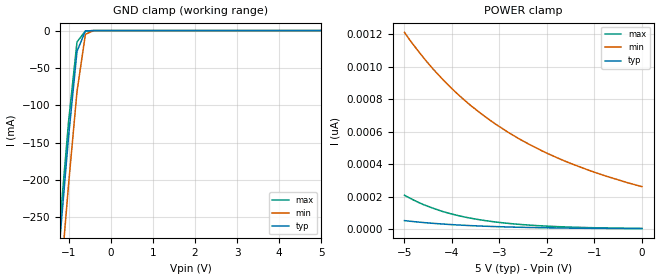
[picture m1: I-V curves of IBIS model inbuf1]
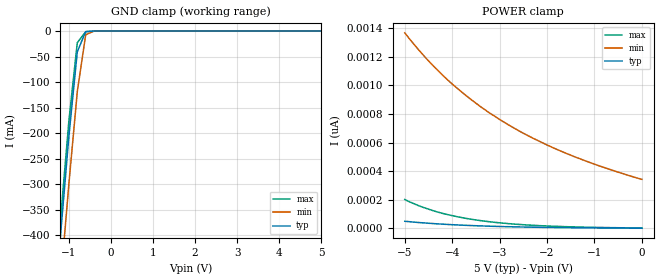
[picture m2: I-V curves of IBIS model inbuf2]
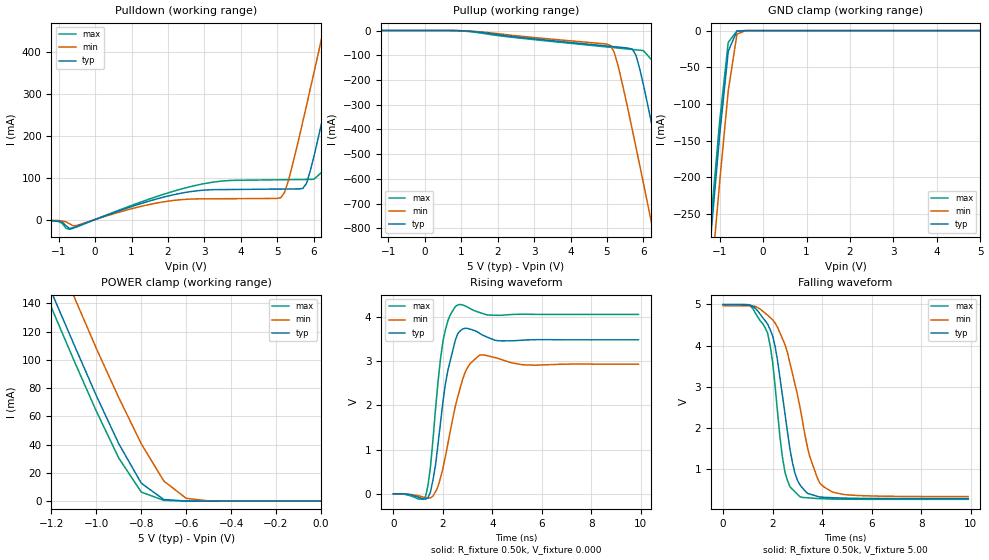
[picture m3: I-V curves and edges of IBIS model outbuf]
| IBIS file 66244l.ibs created by s2ibis2 version 1.0
| North Carolina State University Electronics Research Laboratory  1995
[IBIS ver]   2.1
[File name]   66244l.ibs
[File Rev]   0.1
[Date]   Friday, June 08, 2001
[Source]   IDT
[Notes]   1. Temp typ=25C, min=100C, max=0C 2. Ramp rates based on 500
   ohm load
[Copyright]   Copyright 2001, Integrated Device Technology, Inc.
[Disclaimer] Integrated Device Technology, Inc. ("IDT") hereby grants the
   user of this IBIS model a non-exclusive, nontransferable
   license to use this IBIS model under the following terms.
   The user is granted this license only to use the IBIS model
   and is not granted rights to sell, copy (except as needed to
   run the IBIS model), rent, lease or sub-license the IBIS model
   in whole or in part, or in modified form to anyone.
   The User may modify the IBIS model to suit its specific
   applications, but rights to derivative works and such
   modifications shall belong to IDT.
   This IBIS model is provided on an "AS IS" basis and IDT
   makes absolutely no warranty with respect to the information
   contained herein. IDT DISCLAIMS AND CUSTOMER WAIVES ALL
   WARRANTIES, EXPRESS AND IMPLIED, INCLUDING WARRANTIES OF
   MERCHANTABILITY AND FITNESS FOR A PARTICULAR PURPOSE. THE
   ENTIRE RISK AS TO QUALITY AND PERFORMANCE IS WITH THE
   USER ACCORDINGLY, IN NO EVENT SHALL IDT BE LIABLE
   FOR ANY DIRECT OR INDIRECT DAMAGES, WHETHER IN CONTRACT OR
   TORT, INCLUDING ANY LOST PROFITS OR OTHER INCIDENTAL,
   CONSEQUENTIAL, EXEMPLARY, OR PUNITIVE DAMAGES ARISING OUT OF
   THE USE OR APPLICATION OF THE IBIS model.  Further, IDT
   reserves the right to make changes without notice to any
   product herein to improve reliability, function, or design.
   IDT does not convey any license under patent rights or
   any other intellectual property rights, including those of
   third parties. IDT is not obligated to provide maintenance
   or support for the licensed IBIS model.
|   Component IDT54/74FCT166244T/AT/CT
[Component]   IDT54/74FCT166244T/AT/CT
[Manufacturer]   Integrated Device Technology Inc.
[Package]
| Following package parameters are for SO48-2(TSSOP) package
|[Package]
|| variable   typ   min   max
|R_pkg   15.00m   10.00m   20.00m
|L_pkg   2.30nh   1.40nh   4.50nH
|C_pkg   0.40pF   0.35pF   0.60pF
| Following package parameters are for SO48-1(SSOP), E48-1(CERPAK) packages
| variable   typ   min   max
R_pkg   15.00m   10.00m   20.00m
L_pkg   2.90nH   1.50nH   5.60nH
C_pkg   0.40pF   0.26pF   0.50pF
[Pin]  signal_name   model_name   R_pin   L_pin   C_pin
1   1OEB   inbuf1
2   1Y1   outbuf
3   1Y2   outbuf
4   GND   GND
5   1Y3   outbuf
6   1Y4   outbuf
7   VCC   POWER
8   2Y1   outbuf
9   2Y2   outbuf
10   GND   GND
11   2Y3   outbuf
12   2Y4   outbuf
13   3Y1   outbuf
14   3Y2   outbuf
15   GND   GND
16   3Y3   outbuf
17   3Y4   outbuf
18   VCC   POWER
19   4Y1   outbuf
20   4Y2   outbuf
21   GND   GND
22   4Y3   outbuf
23   4Y4   outbuf
24   4OEB   inbuf1
25   3OEB   inbuf1
26   4A4   inbuf2
27   4A3   inbuf2
28   GND   GND
29   4A2   inbuf2
30   4A1   inbuf2
31   VCC   POWER
32   3A4   inbuf2
33   3A3   inbuf2
34   GND   GND
35   3A2   inbuf2
36   3A1   inbuf2
37   2A4   inbuf2
38   2A3   inbuf2
39   GND   GND
40   2A2   inbuf2
41   2A1   inbuf2
42   VCC   POWER
43   1A4   inbuf2
44   1A3   inbuf2
45   GND   GND
46   1A2   inbuf2
47   1A1   inbuf2
48   2OEB   inbuf1
| Models and submodels in the file (3): inbuf1 (Input), inbuf2 (Input), outbuf (3-state)
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| in   IN1   dummy_model
| oe   OE1   dummy_model
|   Model inbuf1
[Model]   inbuf1
Model_type   Input
Vinl =  0.800V
Vinh =  2.000V
C_comp   3.00pF   NA   NA
[Temperature Range]   25.00   100.00   0.000
[Voltage Range]   5.00V   4.50V   5.50V
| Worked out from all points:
|   GND clamp passes 1 mA (typ) near -0.60 V on its own axis
[GND_clamp]
| voltage   I(typ)   I(min)   I(max)
-5V       -3.018A    -3.076A    -2.999A
-1.4V     -415mA     -480mA     -394mA
-1.2V     -276mA     -341mA     -255mA
-1V       -142mA     -206mA     -122mA
-800mV    -27.87mA   -81.82mA   -15.26mA
-600mV    -480uA     -4.848mA   -551uA
-400mV    -1.016uA   -20.86uA   -873nA
5V        1.855pA    303pA      2.085pA
[POWER_clamp]
| voltage   I(typ)   I(min)   I(max)
-5V       51.46pA    1.212nA    208pA
-4.6V     39.61pA    1.056nA    150pA
-4.4V     34.75pA    987pA      128pA
-4.1V     28.53pA    894pA      99.73pA
-3.9V     25.02pA    837pA      84.6pA
-3.6V     20.53pA    760pA      66.05pA
-3.1V     14.75pA    650pA      43.65pA
-2.8V     12.09pA    593pA      34.01pA
-2.4V     9.265pA    526pA      24.35pA
-1.7V     5.808pA    428pA      13.54pA
-800mV    3.178pA    330pA      6.324pA
0V        1.855pA    261pA      3.199pA
|   Model inbuf2
[Model]   inbuf2
Model_type   Input
Vinl =  0.800V
Vinh =  2.000V
C_comp   3.00pF   NA   NA
[Temperature Range]   25.00   100.00   0.000
[Voltage Range]   5.00V   4.50V   5.50V
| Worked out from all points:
|   GND clamp passes 1 mA (typ) near -0.60 V on its own axis
[GND_clamp]
| voltage   I(typ)   I(min)   I(max)
-5V       -4.387A    -4.471A    -4.36A
-1.4V     -604mA     -698mA     -573mA
-1.2V     -402mA     -496mA     -371mA
-1V       -207mA     -300mA     -177mA
-800mV    -40.8mA    -119mA     -22.8mA
-600mV    -973uA     -7.222mA   -1.303mA
-400mV    -6.41uA    -46.07uA   -11.93uA
5V        1.965pA    393pA      2.176pA
[POWER_clamp]
| voltage   I(typ)   I(min)   I(max)
-5V       50.2pA     1.366nA    202pA
-4.6V     38.73pA    1.207nA    146pA
-4.4V     34.01pA    1.136nA    124pA
-4.1V     27.98pA    1.039nA    97.02pA
-3.6V     20.21pA    900pA      64.36pA
-3.4V     17.74pA    850pA      54.59pA
-3V       13.67pA    761pA      39.26pA
-2.6V     10.54pA    683pA      28.2pA
-2.3V     8.67pA     631pA      22pA
-1.6V     5.503pA    525pA      12.31pA
-900mV    3.5pA      437pA      6.893pA
0V        1.965pA    343pA      3.278pA
|   Model outbuf
[Model]   outbuf
Model_type   3-state
Polarity   Non-Inverting
Enable   Active-High
Vinl =  0.800V
Vinh =  2.000V
C_comp   3.00pF   NA   NA
[Temperature Range]   25.00   100.00   0.000
[Voltage Range]   5.00V   4.50V   5.50V
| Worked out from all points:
|   slope of the pulldown table from 0 to 0.75 V, typ, clamps not added: 32 ohm
|   slope of the pullup table from 0 to 0.75 V, typ, clamps not added: 16.9 kohm
|   GND clamp passes 1 mA (typ) near -0.60 V on its own axis
|   POWER clamp passes 1 mA (typ) near -0.69 V on its own axis
|   rising waveform, R_fixture 0.50k, V_fixture 0.000: 20-80 % time 487ps typ, 670ps min, 420ps max; typ from 0 V to 3.49 V
|   falling waveform, R_fixture 0.50k, V_fixture 5.00: 20-80 % time 708ps typ, 1.04ns min, 535ps max; typ from 5 V to 0.294 V
[Pulldown]
| voltage   I(typ)   I(min)   I(max)
-5V       0A         0A         0A
-1.4V     -1.4mA     -1.2mA     -1.5mA
-700mV    -21.48mA   -10.28mA   -23.37mA
2.4V      63.27mA    47.55mA    73.49mA
5.1V      72.54mA    52.22mA    94.74mA
5.3V      72.68mA    90.95mA    94.95mA
5.8V      85.74mA    270mA      95.45mA
6.4V      298mA      503mA      126mA
6.8V      454mA      660mA      272mA
7.2V      613mA      818mA      428mA
7.6V      772mA      977mA      586mA
10V       1.734A     1.934A     1.549A
[Pullup]
| voltage   I(typ)   I(min)   I(max)
-5V       0A         0A         0A
900mV     -315uA     -296uA     -632uA
5V        -62.63mA   -55.04mA   -66.48mA
5.2V      -65.46mA   -88.64mA   -69.4mA
5.7V      -75.8mA    -405mA     -76.67mA
5.8V      -102mA     -475mA     -78.12mA
6V        -219mA     -617mA     -81.11mA
6.4V      -498mA     -906mA     -148mA
6.8V      -787mA     -1.197A    -417mA
7.2V      -1.079A    -1.49A     -705mA
7.6V      -1.373A    -1.784A    -998mA
10V       -3.151A    -3.558A    -2.774A
[GND_clamp]
| voltage   I(typ)   I(min)   I(max)
-5V       -3.126A    -3.162A    -3.124A
-1.4V     -422mA     -485mA     -404mA
-1.2V     -280mA     -344mA     -261mA
-1V       -144mA     -208mA     -125mA
-800mV    -28.18mA   -82.09mA   -16.01mA
-600mV    -487uA     -4.87mA    -593uA
-400mV    -1.041uA   -20.98uA   -995nA
5V        1.911pA    145uA      2.071pA
[POWER_clamp]
| voltage   I(typ)   I(min)   I(max)
-5V       1.658A     1.682A     1.65A
-1.3V     186mA      220mA      175mA
-1.2V     148mA      182mA      137mA
-1.1V     111mA      145mA      99.7mA
-1V       74.62mA    108mA      63.64mA
-900mV    40.55mA    73.19mA    30.44mA
-800mV    12.71mA    40.62mA    6.427mA
-700mV    1.113mA    14.29mA    552uA
-600mV    55.94uA    1.985mA    66.61uA
-500mV    1.923uA    144uA      3.688uA
0V        1.911pA    260pA      3.223pA
[Ramp]
| variable   typ   min   max
dV/dt_r   2.09/0.49n   1.76/0.67n   2.44/0.42n
dV/dt_f   2.82/0.71n   2.52/1.02n   3.12/0.54n
R_load = 0.50k
[Rising Waveform]
R_fixture = 0.50k
V_fixture = 0.000
| time   V(typ)   V(min)   V(max)
0s        0V         0V         0V
1.3ns     -121mV     -88.65mV   -60.88mV
1.5ns     42.72mV    -93.72mV   620mV
1.6ns     317mV      -50.98mV   1.228V
1.8ns     1.107V     161mV      2.515V
2ns       2.073V     572mV      3.447V
2.5ns     3.474V     1.973V     4.238V
2.9ns     3.75V      2.753V     4.255V
3.5ns     3.627V     3.142V     4.102V
9.9ns     3.487V     2.935V     4.063V
[Falling Waveform]
R_fixture = 0.50k
V_fixture = 5.00
| time   V(typ)   V(min)   V(max)
0s        5V         4.97V      5V
1.1ns     4.987V     4.968V     4.961V
1.9ns     4.392V     4.684V     4.006V
2.1ns     3.985V     4.552V     3.029V
2.5ns     2.348V     4.029V     929mV
2.8ns     1.169V     3.327V     519mV
3.1ns     628mV      2.528V     340mV
3.8ns     349mV      806mV      295mV
4.4ns     315mV      456mV      282mV
9.9ns     294mV      341mV      275mV
